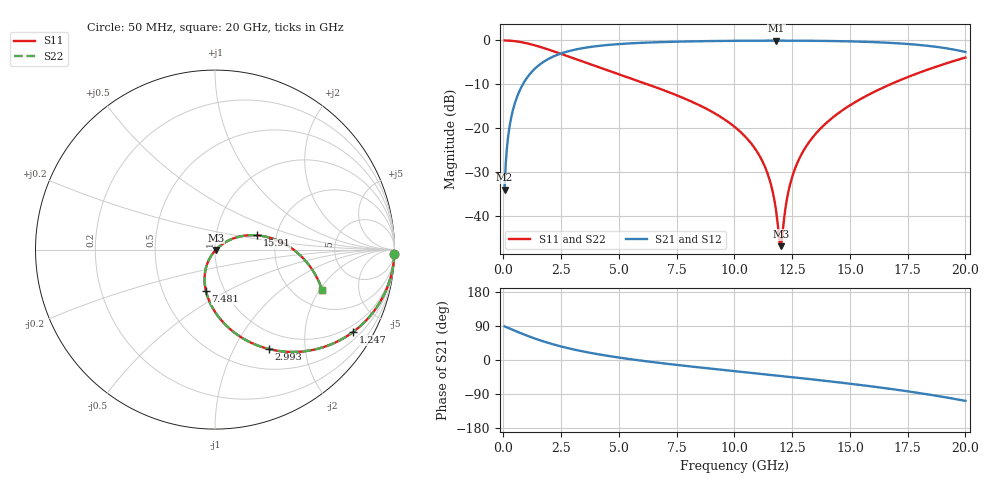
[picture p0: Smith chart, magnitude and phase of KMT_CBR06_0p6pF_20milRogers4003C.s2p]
! Data measured by Modelithics Inc. support@modelithics.com 813-866-6335
! KEMET CBR0603 0.6pF, Pad Width= 0.851mm, Pad Length= 0.64mm, Pad Gap= 0.62mm, 20mil Rogers 4003C substrate Data, January 2022
# hz S ma R 50
! 2 Port Network Data from SP1.SP block
! freq  magS11  angS11  magS21  angS21  magS12  angS12  magS22  angS22
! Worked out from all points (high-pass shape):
!   401 points, 50 MHz to 20 GHz, reference 50 ohm
!   highest |S21| = -0.04 dB at 11.82 GHz (marker M1); lowest = -34.1 dB at 50 MHz (marker M2)
!   |S21| within 3 dB of the highest: 2.459 GHz to end of sweep
!   lowest |S11| = -47.0 dB at 12.02 GHz (marker M3), VSWR 1.01, Z = 50.4 - j0.219 ohm
!   |S11| at or under -10 dB: 6.234 GHz to 16.76 GHz (10.53 GHz wide, 91.6 % of centre)
!   |S22| runs from -47.0 to 0.0 dB; largest |S21 - S12| = 0
!   S11 on the Smith chart (normalised r, x): 50 MHz: 1, -87; 1.247 GHz: 0.75, -3.48; 2.993 GHz: 0.76, -1.39; 7.481 GHz: 0.82, -0.40; 15.91 GHz: 1.59, +0.27; 20 GHz: 2.78, -2.11
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5e7  0.9998 -1.3  0.01976 88.7  0.01976 88.7  0.9998 -1.3
2.495e8  0.9951 -6.5  0.09816 83.5  0.09816 83.5  0.9951 -6.5
4.49e8  0.9845 -11.7  0.1749 78.3  0.1749 78.3  0.9845 -11.7
7.98125e8  0.9533 -20.4  0.3014 69.6  0.3014 69.6  0.9533 -20.4
1.247e9  0.8956 -30.8  0.444 59.1  0.444 59.1  0.8956 -30.8
2.992625e9  0.6312 -61.4  0.7738 28.4  0.7738 28.4  0.6312 -61.4
3.391625e9  0.579 -66.6  0.8134 23.2  0.8134 23.2  0.579 -66.6
6.73325e9  0.2832 -97.0  0.9561 -7.5  0.9561 -7.5  0.2832 -97.0
7.481375e9  0.2377 -102.2  0.9682 -12.8  0.9682 -12.8  0.2377 -102.2
1.0025e10  0.1024 -117.5  0.9909 -29.5  0.9909 -29.5  0.1024 -117.5
1.1222e10  0.04127 -121.6  0.9948 -37.1  0.9948 -37.1  0.04127 -121.6
1.157112e10  0.02322 -119.1  0.9952 -39.3  0.9952 -39.3  0.02322 -119.1
1.18205e10  0.01055 -107.1  0.9953 -40.9  0.9953 -40.9  0.01055 -107.1
1.192025e10  0.006106 -86.7  0.9953 -41.6  0.9953 -41.6  0.006106 -86.7
1.202e10  0.004482 -29.0  0.9952 -42.2  0.9952 -42.2  0.004482 -29.0
1.231925e10  0.01786 31.2  0.9949 -44.2  0.9949 -44.2  0.01786 31.2
1.251875e10  0.02865 35.2  0.9945 -45.5  0.9945 -45.5  0.02865 35.2
1.336662e10  0.07703 35.0  0.9914 -51.1  0.9914 -51.1  0.07703 35.0
1.591025e10  0.2479 18.7  0.96 -69.4  0.96 -69.4  0.2479 18.7
1.670825e10  0.3119 12.3  0.9395 -75.8  0.9395 -75.8  0.3119 12.3
1.8404e10  0.4681 -3.1  0.8665 -91.0  0.8665 -91.0  0.4681 -3.1
2e10  0.638 -20.7  0.7378 -107.8  0.7378 -107.8  0.638 -20.7
